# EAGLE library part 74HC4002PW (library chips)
NOR Gate IC 2 Channel 14-TSSOP
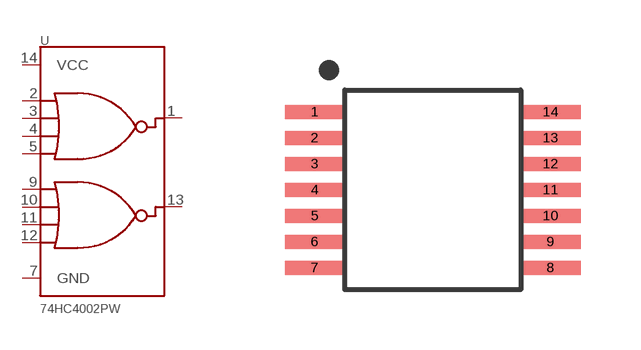
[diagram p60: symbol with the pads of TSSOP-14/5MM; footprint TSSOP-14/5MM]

Designator prefix U

## 74HC4002PW (DIGIKEY: 568-8879-1-ND)  [TSSOP-14/5MM]
1  AOUT
2  A1
3  A2
4  A3
5  A4
7  GND
9  B1
10  B2
11  B3
12  B4
13  BOUT
14  VCC

## Footprint TSSOP-14/5MM (pad centres in mm)
smd 1.5 x 0.35: 1 -2.95,1.95; 2 -2.95,1.3; 3 -2.95,0.65; 4 -2.95,0; 5 -2.95,-0.65; 6 -2.95,-1.3; 7 -2.95,-1.95; 8 2.95,-1.95; 9 2.95,-1.3; 10 2.95,-0.65; 11 2.95,0; 12 2.95,0.65; 13 2.95,1.3; 14 2.95,1.95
